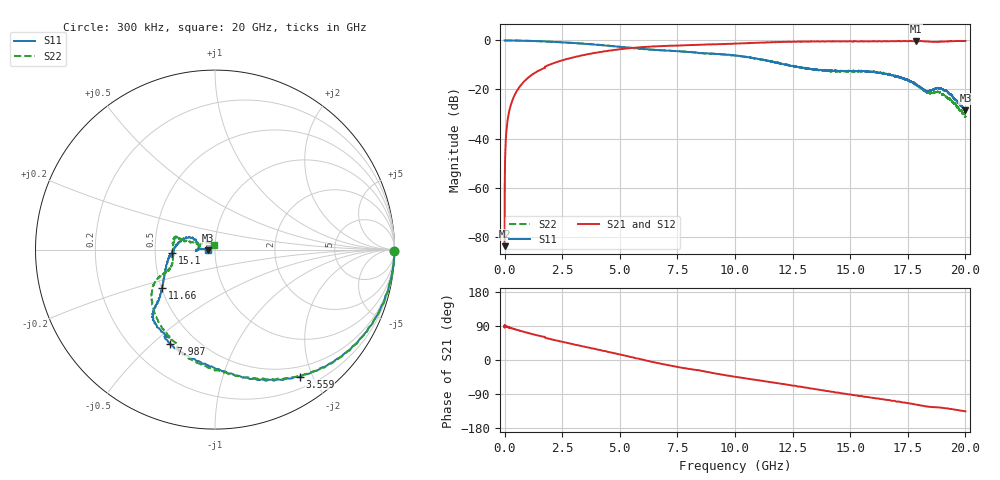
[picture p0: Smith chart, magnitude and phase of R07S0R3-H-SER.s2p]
!{R07S0R3}
!Johanson Technology Inc.
!www.johansontechnology.com
!Test Board Conditions:
!Substrate Type  RO4350B
!Substrate Thickness  10 mil
!Substrate Dk  3.66
!TL Type: GCPW
!TL Trace Width  21 mil
!TL Gap  20 mil
!Electrode orientation  Horizontal
!DUT TOPOLOGY	SERIES
!Mounting Pad LxW  16x21 mil
! Created Fri Feb  5 23:01:43 2021
# hz S ma R 50
! 2 Port Network Data from SP1.SP block
! freq  magS11  angS11  magS21  angS21  magS12  angS12  magS22  angS22
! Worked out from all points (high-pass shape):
!   20001 points, 300 kHz to 20 GHz, reference 50 ohm
!   highest |S21| = -0.18 dB at 17.84 GHz (marker M1); lowest = -83.9 dB at 300 kHz (marker M2)
!   |S21| within 3 dB of the highest: 5.411203 GHz to 5.411359 GHz (155.9 kHz wide, 0.00288 % of centre); 5.419 GHz to end of sweep
!   lowest |S11| = -28.5 dB at 20 GHz (marker M3), VSWR 1.08, Z = 46.4 - j0.266 ohm
!   |S11| at or under -10 dB: 12.22518 GHz to 12.22659 GHz (1.418 MHz wide, 0.0116 % of centre); 12.25144 GHz to 12.25928 GHz (7.846 MHz wide, 0.064 % of centre); 12.26 GHz to end of sweep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
!   |S22| runs from -31.3 to 0.0 dB; largest |S21 - S12| = 0.013
!   S11 on the Smith chart (normalised r, x): 300 kHz: open; 3.559 GHz: 0.36, -1.82; 7.987 GHz: 0.36, -0.57; 11.66 GHz: 0.50, -0.25; 15.1 GHz: 0.62, -0.03; 20 GHz: 0.93, -0.01
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300000  0.9993 -0.6  6.376e-05 87.0  9.151e-05 100.1  1 -0.5
1.023e8  0.9972 -1.9  0.01833 88.0  0.01841 88.1  0.9968 -1.9
1.393e8  0.9987 -2.6  0.02519 87.0  0.02512 87.3  0.9993 -2.6
2.783e8  0.9976 -5.2  0.04991 84.4  0.0499 84.3  0.9968 -5.2
5.153e8  0.9953 -9.5  0.09059 80.0  0.09055 80.0  0.9952 -9.6
1.0063e9  0.9828 -17.8  0.1716 71.6  0.1713 71.6  0.9822 -18.1
1.8503e9  0.9472 -32.4  0.3067 57.1  0.3055 57.2  0.9481 -32.8
3.3343e9  0.8658 -53.2  0.4937 36.8  0.4927 36.8  0.8681 -52.7
3.5593e9  0.8506 -56.2  0.5187 33.8  0.5189 33.9  0.8528 -55.5
5.0333e9  0.7406 -75.4  0.6642 14.3  0.6639 14.4  0.7377 -75.1
6.6673e9  0.6383 -96.4  0.7639 -8.3  0.7639 -8.2  0.6367 -99.6
7.9873e9  0.5821 -115.3  0.8027 -23.5  0.8026 -23.4  0.5858 -111.0
1.00003e10  0.4961 -134.3  0.8604 -44.2  0.8618 -44.1  0.4897 -133.3
1.16633e10  0.3635 -143.9  0.9203 -59.3  0.9219 -59.3  0.3671 -152.5
1.33343e10  0.2599 -170.4  0.9549 -75.4  0.9555 -75.4  0.2595 -158.9
1.51043e10  0.238 -175.4  0.9463 -92.1  0.9542 -92.5  0.2355 170.4
1.66673e10  0.1999 167.7  0.9625 -105.8  0.9644 -105.8  0.2078 162.6
1.78423e10  0.1287 155.6  0.9796 -117.5  0.9774 -117.0  0.1255 161.9
1.83293e10  0.09191 170.3  0.955 -122.7  0.9547 -122.6  0.08752 167.8
1.91103e10  0.09442 179.1  0.9531 -127.1  0.9522 -126.9  0.07359 152.1
1.99993e10  0.0374 -175.6  0.9773 -135.5  0.9774 -135.5  0.02777 105.8
2e10  0.03746 -174.6  0.9759 -135.5  0.9763 -135.5  0.02708 106.3
